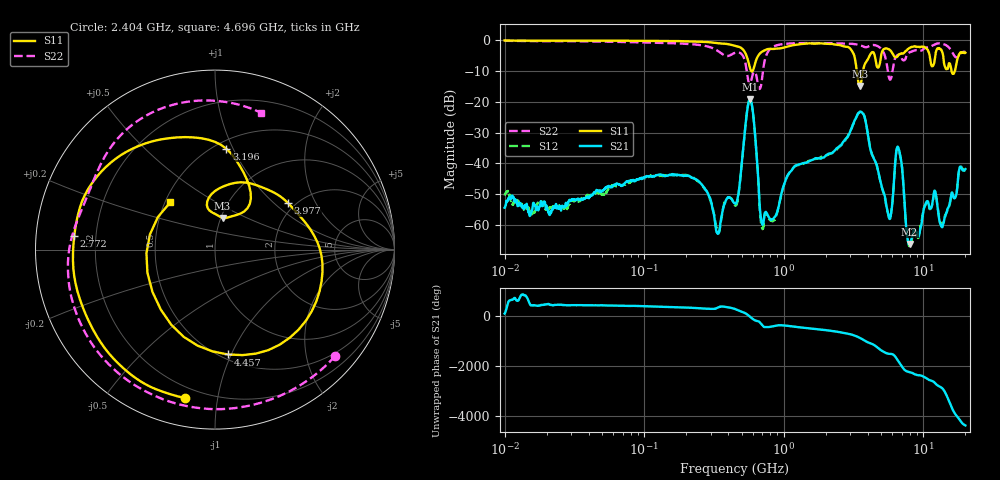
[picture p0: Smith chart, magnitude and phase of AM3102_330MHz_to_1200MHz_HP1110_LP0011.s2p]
! Date/Time: Tue, Sep 11, 2018 5:23 PM
! Network Analyzer: Agilent Technologies E8362B Rev: A.07.50.63
! Sweep from 0.010 to 20.000 GHz, 1601 Points, Sweep Type: LOG
! Power Supply: 4.949 V, 0.001 A
# Hz S DB R 50
!freq MagS11 AngS11 MagS21 AngS21 MagS12 AngS12 MagS22 AngS22
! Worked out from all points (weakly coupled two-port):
!   1601 points, 10 MHz to 20 GHz, reference 50 ohm
!   highest |S21| = -19.19 dB at 572.5 MHz (marker M1); lowest = -66.3 dB at 7.958 GHz (marker M2)
!   lowest |S11| = -14.8 dB at 3.498 GHz (marker M3), VSWR 1.44, Z = 50.9 + j18.6 ohm
!   |S11| at or under -10 dB: 584.4 MHz to 597.4 MHz (12.97 MHz wide, 2.2 % of centre); 3.338 GHz to 3.693 GHz (355.4 MHz wide, 10.1 % of centre); 15.92 GHz to 16.8 GHz (880.8 MHz wide, 5.38 % of centre)
!   |S22| runs from -15.8 to -0.2 dB; largest |S21 - S12| = 0.0059
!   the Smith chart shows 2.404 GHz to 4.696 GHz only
!   S11 on the Smith chart (normalised r, x): 2.404 GHz: 0.14, -0.81; 2.772 GHz: 0.12, +0.05; 3.196 GHz: 0.57, +0.94; 3.977 GHz: 1.82, +1.24; 4.457 GHz: 0.54, -0.97; 4.696 GHz: 0.53, +0.32
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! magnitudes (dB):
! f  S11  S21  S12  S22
! 10 MHz  0.0  -54.5  -50.5  -0.2
! 35.55 MHz  -0.1  -51.8  -51.3  -0.3
! 126.4 MHz  -0.2  -43.8  -44.1  -0.8
! 248.1 MHz  -0.5  -46.0  -46.1  -1.5
! 336.3 MHz  -0.9  -63.0  -62.3  -3.4
! 447.2 MHz  -1.8  -53.0  -53.7  -4.1
! 572.5 MHz  -9.0  -19.2  -19.3  -14.1
! 699 MHz  -3.7  -59.6  -61.2  -12.5
! 1.59 GHz  -1.0  -38.9  -38.9  -0.9
! 2.404 GHz  -1.5  -35.0  -35.5  -1.0
! 2.772 GHz  -2.1  -32.1  -32.4  -1.0
! 3.196 GHz  -4.9  -26.3  -26.4  -1.2
! 3.498 GHz  -14.8  -23.4  -23.3  -1.6
! 3.977 GHz  -6.3  -30.0  -29.8  -2.1
! 4.457 GHz  -4.6  -38.9  -38.7  -1.5
! 4.696 GHz  -8.8  -41.7  -41.8  -1.9
! 5.652 GHz  -2.9  -57.3  -57.6  -11.9
! 6.643 GHz  -4.7  -35.2  -35.3  -4.7
! 7.958 GHz  -2.5  -66.3  -67.0  -3.9
! 12.03 GHz  -6.6  -48.9  -49.3  -1.4
! 13.68 GHz  -3.9  -60.8  -60.0  -1.1
! 20 GHz  -4.1  -41.9  -42.4  -3.7
